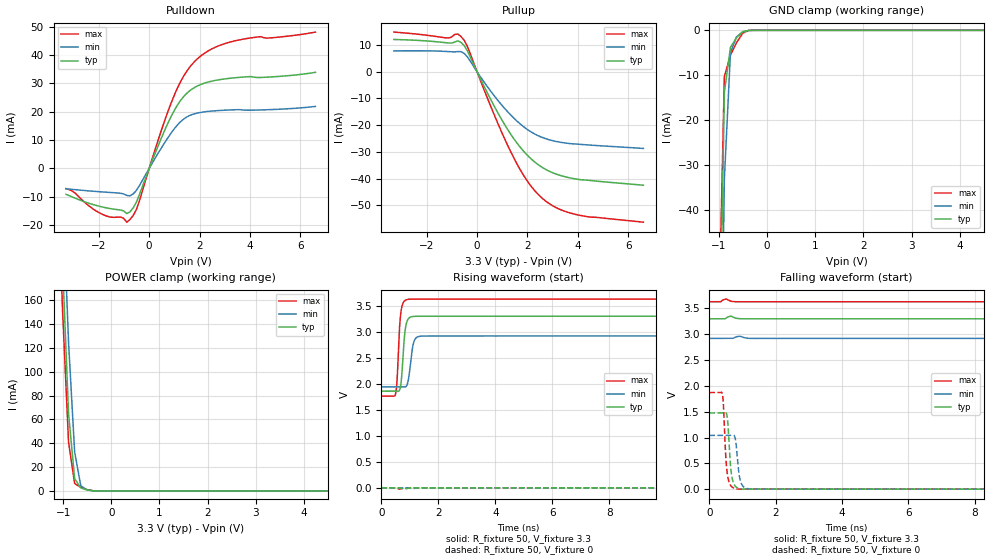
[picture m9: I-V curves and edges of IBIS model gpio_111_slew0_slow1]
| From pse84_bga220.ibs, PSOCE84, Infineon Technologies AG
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[Model] gpio_111_slew0_slow1
Model_type I/O
Enable   Active-High
Vinl  =  0.99
Vinh  =  2.31
Vmeas =  1.65
Cref  =  15e-12
| Capacitance   typ   min   max
C_comp   1.09946e-12   1.08623e-12   1.11440e-12
| Variables   typ   min   max
[GND Clamp Reference]   0   0   0
[POWER Clamp Reference]   3.3   2.92   3.63
[Pulldown Reference]   0   0   0
[Pullup Reference]   3.3   2.92   3.63
[Temperature Range]   25   125   -40
[Voltage Range]   3.3   2.92   3.63
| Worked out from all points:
|   slope of the pulldown table from 0 to 0.495 V, typ, clamps not added: 45.2 ohm
|   slope of the pullup table from 0 to 0.495 V, typ, clamps not added: 52.1 ohm
|   GND clamp passes 1 mA (typ) near -0.57 V on its own axis
|   POWER clamp passes 1 mA (typ) near -0.52 V on its own axis
|   falling waveform, R_fixture 50, V_fixture 3.3: 20-80 % time 625ns typ, 958ns min, 328ns max; typ from 3.3 V to 1.86 V
|   falling waveform, R_fixture 50, V_fixture 0: 20-80 % time 96.4ps typ, 105ps min, 91.5ps max; typ from 1.48 V to 0 V
|   rising waveform, R_fixture 50, V_fixture 3.3: 20-80 % time 117ps typ, 138ps min, 103ps max; typ from 1.86 V to 3.3 V
|   rising waveform, R_fixture 50, V_fixture 0: 20-80 % time 609ns typ, 904ns min, 366ns max; typ from 0 V to 1.47 V
[GND Clamp]
| Voltage   I(typ)   I(min)   I(max)
-1.65V    -892.5mA   -911.9mA   -883.9mA
-1.015V   -92.32mA   -129.7mA   -71.28mA
-888.3mV  -13.83mA   -33.21mA   -10.31mA
-761.4mV  -3.792mA   -4.944mA   -5.509mA
-634.5mV  -1.622mA   -1.436mA   -2.707mA
-507.6mV  -326.2uA   -352.3uA   -651.6uA
-380.7mV  -13.48uA   -32.14uA   -19.55uA
-253.8mV  -189.4nA   -1.276uA   -466.7nA
6.6V      0A         0A         0A
[POWER Clamp]
| Voltage   I(typ)   I(min)   I(max)
-1.523V   838.1mA    872.9mA    823.9mA
-1.142V   346.5mA    405.1mA    310.5mA
-1.015V   193mA      257.4mA    153.9mA
-888.3mV  64.97mA    124.9mA    40.96mA
-761.4mV  10.28mA    32.7mA     6.184mA
-634.5mV  2.553mA    4.346mA    3.067mA
-507.6mV  805.9uA    960.7uA    1.159mA
-253.8mV  1.454uA    10.02uA    1.678uA
6.6V      0A         0A         0A
[Pulldown]
| Voltage   I(typ)   I(min)   I(max)
-3.3V     -9.135mA   -7.157mA   -7.087mA
-2.03V    -13.19mA   -8.152mA   -15.36mA
-1.142V   -14.64mA   -8.738mA   -17.11mA
-888.3mV  -15.9mA    -9.489mA   -18.93mA
-507.6mV  -11.91mA   -7.751mA   -14.53mA
455.2mV   10.12mA    6.824mA    12.65mA
1.024V    20.87mA    14.3mA     26.39mA
1.366V    25.31mA    17.39mA    32.51mA
1.821V    28.65mA    19.34mA    37.87mA
2.503V    30.82mA    20.26mA    42.24mA
3.3V      31.89mA    20.67mA    44.77mA
6.6V      33.91mA    21.88mA    48.09mA
[Pullup]
| Voltage   I(typ)   I(min)   I(max)
-3.3V     12.1mA     7.82mA     14.87mA
-1.142V   10.79mA    7.573mA    12.65mA
-761.4mV  11.61mA    7.566mA    14.12mA
-634.5mV  10.98mA    7.55mA     13.18mA
-380.7mV  7.78mA     5.549mA    9.437mA
682.8mV   -12.9mA    -9.017mA   -16.15mA
1.479V    -25.35mA   -17.53mA   -32.65mA
2.048V    -31.76mA   -21.95mA   -41.65mA
2.731V    -36.61mA   -25.08mA   -48.5mA
3.3V      -38.82mA   -26.38mA   -51.59mA
4.051V    -40.35mA   -27.14mA   -53.71mA
6.6V      -42.49mA   -28.71mA   -56.34mA
[Ramp]
dV/dt_r   0.882956/0.609094u  0.617386/0.904453u  1.12272/0.36647u
dV/dt_f   0.863955/0.625008u  0.58199/0.958406u  1.12003/0.328447u
R_load = 50
[Falling Waveform]
R_fixture = 50
V_fixture = 3.3
V_fixture_min = 2.92
V_fixture_max = 3.63
| Time   V(typ)   V(min)   V(max)
0s        3.3V       2.92V      3.63V
120.7ns   3.3V       2.92V      3.577V
223.3ns   3.264V     2.92V      3.057V
303.9ns   3.119V     2.913V     2.677V
426.1ns   2.842V     2.853V     2.298V
589ns     2.537V     2.702V     2.048V
792.6ns   2.286V     2.514V     1.909V
1.185us   2.052V     2.265V     1.81V
1.837us   1.919V     2.075V     1.772V
4us       1.86V      1.95V      1.763V
[Falling Waveform]
R_fixture = 50
V_fixture = 0
V_fixture_min = 0
V_fixture_max = 0
| Time   V(typ)   V(min)   V(max)
0s        1.475V     1.041V     1.872V
390.3ps   1.475V     1.041V     1.848V
427.4ps   1.475V     1.041V     1.599V
516.6ps   1.464V     1.041V     441.2mV
553.3ps   1.318V     1.041V     250.8mV
682.6ps   227.9mV    1.042V     42.28mV
782.2ps   57.34mV    979.2mV    9.038mV
889.4ps   13.56mV    324.7mV    487.8uV
958.2ps   4.163mV    119mV      54.38uV
4us       16.19nV    462.9nV    7.796nV
[Rising Waveform]
R_fixture = 50
V_fixture = 3.3
V_fixture_min = 2.92
V_fixture_max = 3.63
| Time   V(typ)   V(min)   V(max)
0s        1.858V     1.94V      1.763V
493.1ps   1.858V     1.94V      1.8V
548.4ps   1.858V     1.94V      2.062V
636.7ps   1.88V      1.94V      3.092V
714ps     2.163V     1.94V      3.474V
847.5ps   3.086V     1.943V     3.61V
1.088ns   3.294V     2.687V     3.629V
1.378ns   3.299V     2.916V     3.628V
5.698ns   3.3V       2.92V      3.63V
4us       3.3V       2.92V      3.63V
[Rising Waveform]
R_fixture = 50
V_fixture = 0
V_fixture_min = 0
V_fixture_max = 0
| Time   V(typ)   V(min)   V(max)
0s        13.96nV    450.5nV    8.038nV
129.9ns   526uV      140.7uV    75.54mV
225.4ns   54.7mV     2.725mV    461.3mV
339.3ns   253.3mV    34.25mV    938.7mV
502.2ns   588.6mV    153.8mV    1.385V
624.4ns   806.8mV    268.2mV    1.56V
828ns     1.066V     455.5mV    1.705V
1.186us   1.283V     705.3mV    1.806V
1.814us   1.409V     908.8mV    1.854V
4us       1.472V     1.029V     1.871V
